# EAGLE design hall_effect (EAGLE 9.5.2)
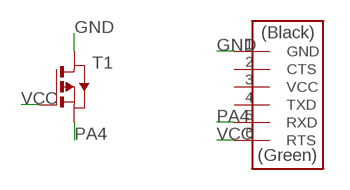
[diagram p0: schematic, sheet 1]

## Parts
T1  MOSFET_PSOT23  [SOT-23]
U$1  CONN_06_FTDI-SMD-HEADER  [1X06SMD]

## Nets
GND: T1.1(D) U$1.1(GND)
PA4: T1.2(S) U$1.5(RXD)
VCC: T1.3(G) U$1.6(RTS)
Unconnected: U$1.2(CTS) U$1.3(VCC) U$1.4(TXD)

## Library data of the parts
T1 = fab:MOSFET_P: MOS FET
U$1 = fab:CONN_06_FTDI-SMD-HEADER

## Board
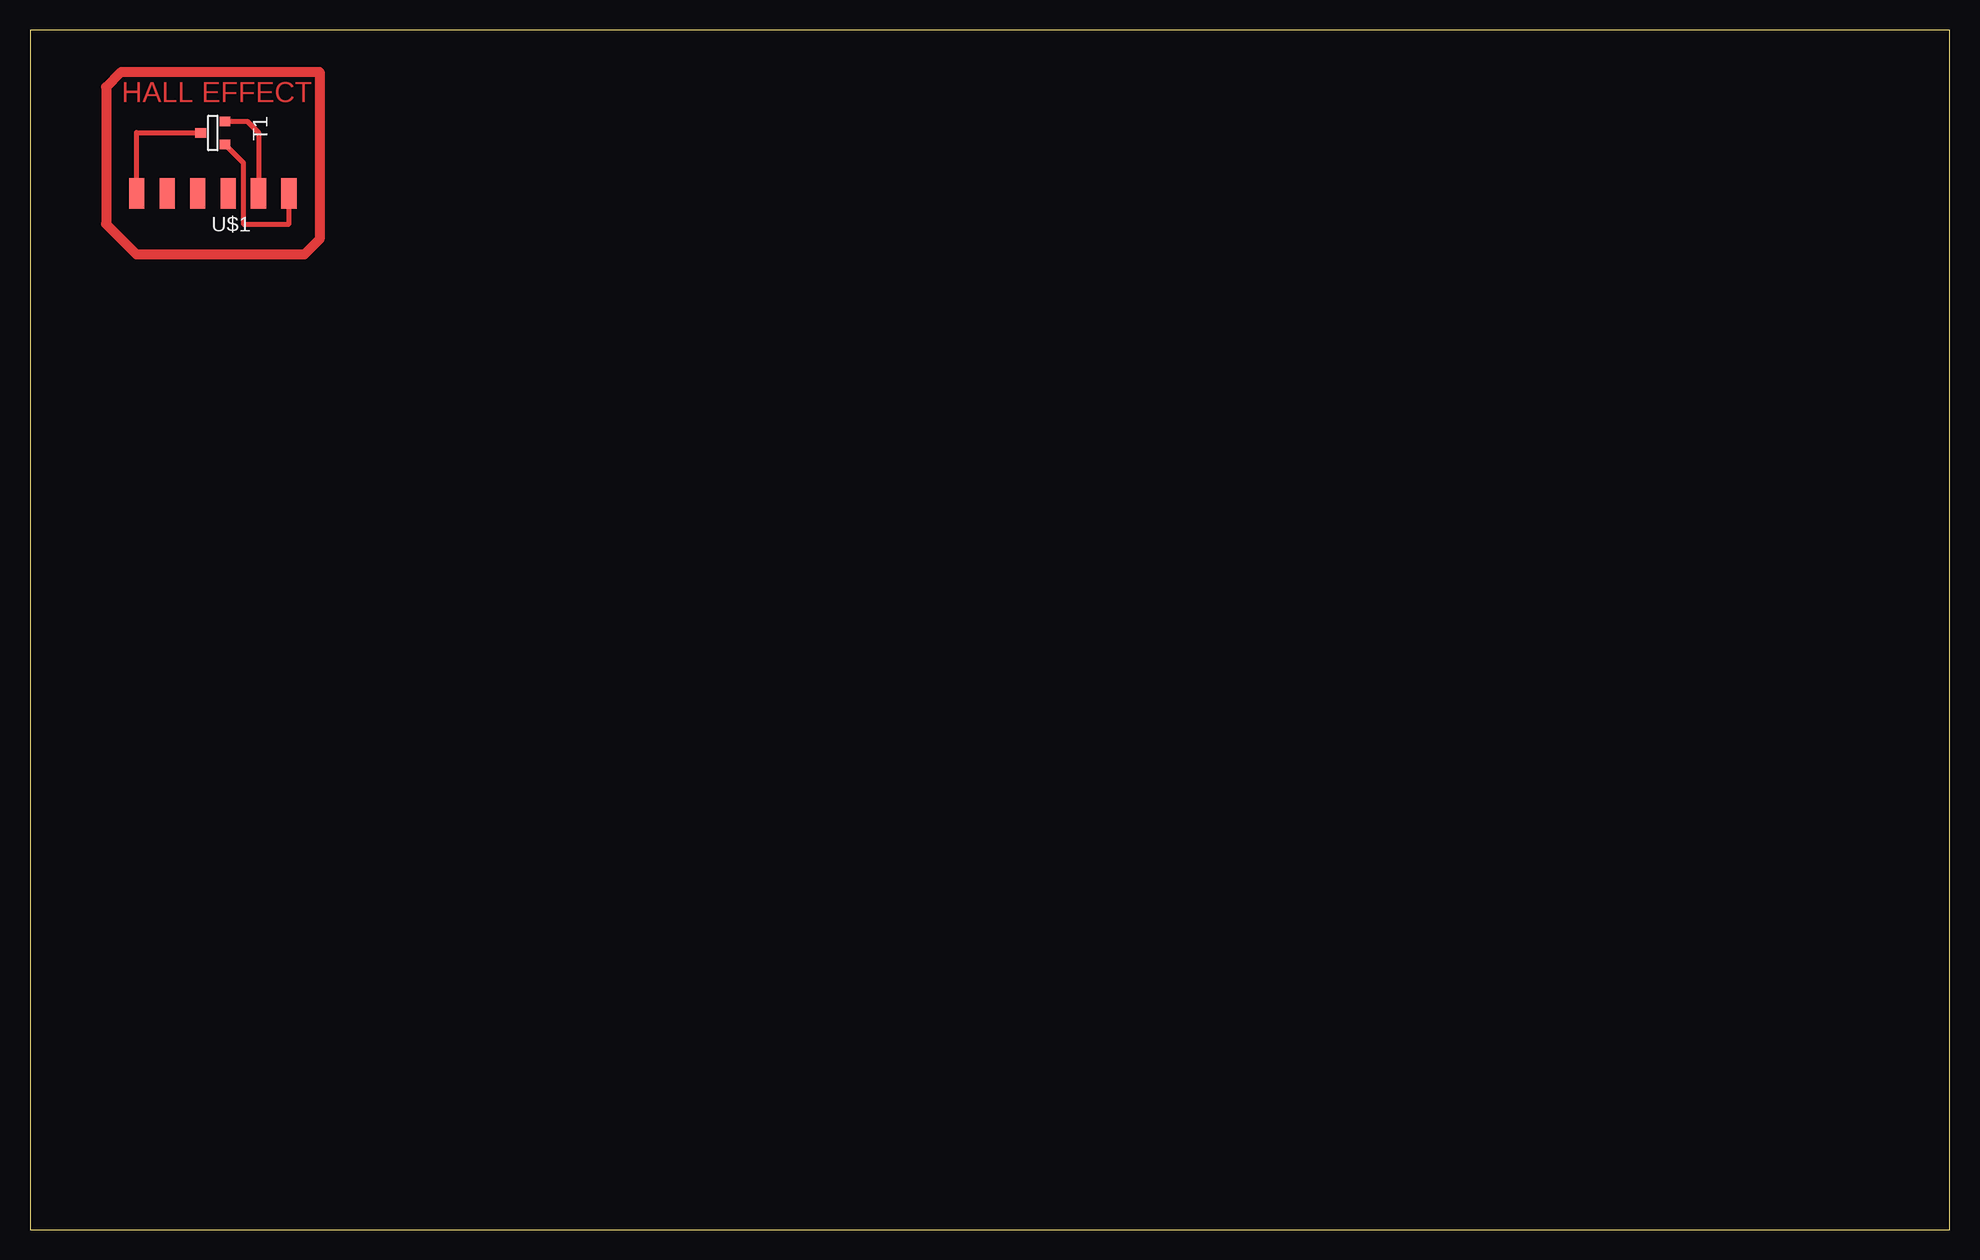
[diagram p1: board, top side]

Size 160 x 100 mm. Coordinates in mm from the lower left corner, seen from the top.
Outline: 0,0 160,0 160,100 0,100 0,0
Copper layers (1*16): Top 0.035mm / dielectric 1.5mm / Bottom 0.035mm
Design rules "default": minimum track width 6mil, minimum drill 0.35mm, track to track 6mil, track to pad 6mil, pad to pad 6mil, via to via 6mil, smd to smd 6mil, copper to edge 40mil, drill to drill 6mil, minimum pad ring 10mil, minimum via ring 8mil, stop-mask expansion 4mil, vias tented up to drill 0mil, thermal gap 10mil

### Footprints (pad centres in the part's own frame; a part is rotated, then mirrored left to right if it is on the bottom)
SOT-23 = smd 0.787 x 0.889: 1 0.025,-1.016; 2 -0.94,1.016; 3 0.991,1.016
1X06SMD = smd 2.54 x 1.27: 1 0,6.35; 2 0,3.81; 3 0,1.27; 4 0,-1.27; 5 0,-3.81; 6 0,-6.35

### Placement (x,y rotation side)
T1  15.24,91.44 270 top
U$1  15.24,86.36 90 top

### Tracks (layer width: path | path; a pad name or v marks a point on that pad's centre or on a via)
GND
  Top 0.406: U$1.1 8.89,91.44 14.2,91.44 T1.1
N$2
  Top 0.813: 6.35,95.25 7.62,96.52 24.13,96.52 24.13,82.55 22.86,81.28 8.89,81.28 6.35,83.82 6.35,95.25
PA4
  Top 0.406: T1.2 18.11,92.38 19.05,91.44 U$1.5
VCC
  Top 0.406: T1.3 17.78,88.92 17.78,83.82 21.59,83.82 U$1.6

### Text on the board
Top: HALL EFFECT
